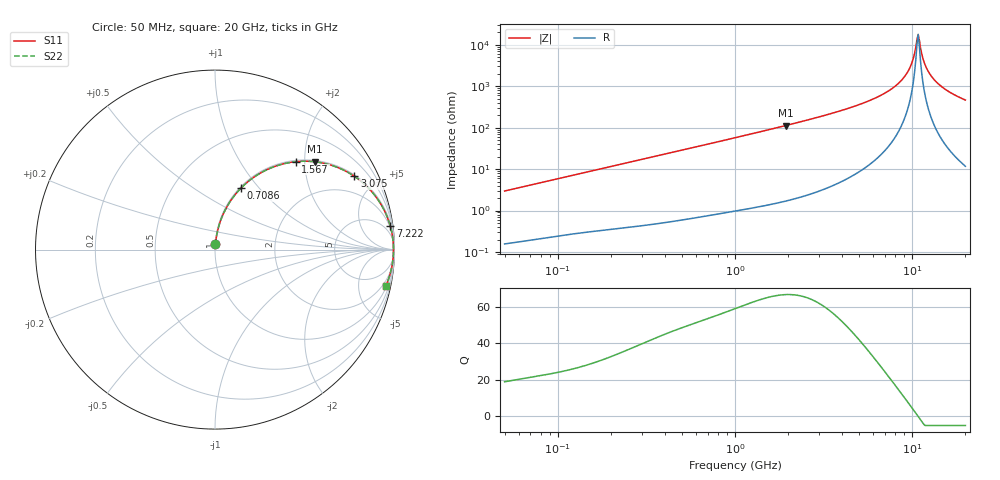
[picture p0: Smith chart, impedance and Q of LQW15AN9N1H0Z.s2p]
!Murata Part Number: LQW15AN9N1H0Z
!These Parameters are Measured in Series Mode Connection
!  o--[Z]--o
!Port1  Port2
!  o-------o
!Freq. Start=50[MHz] Stop=20[GHz], 401[Steps]
# Hz S RI R 50
!Freq.(Hz) S11(Real) S11(Imag) S21(Real) S21(Imag) S12(Real) S12(Imag) S22(Real) S22(Imag)
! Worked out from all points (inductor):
!   401 points, 50 MHz to 20 GHz, reference 50 ohm
!   read as one part in series: L = 9.38 nH near 51.52 MHz
!   highest Q = 66.6 at 1.933 GHz (marker M1), where L = 9.27 nH
!   self-resonance near 10.66 GHz
!   S11 on the Smith chart (normalised r, x): 50 MHz: 1.00, +0.06; 708.6 MHz: 1.02, +0.81; 1.567 GHz: 1.03, +1.81; 3.075 GHz: 1.06, +3.77; 7.222 GHz: 2, +15; 20 GHz: 1.23, -9.29
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5e7  0.00243 0.0295  0.9976 -0.0295  0.9976 -0.0295  0.00243 0.0295
1.364002e8  0.00906 0.0781  0.9909 -0.0781  0.9909 -0.0781  0.00906 0.0781
3.721004e8  0.0476 0.2017  0.9524 -0.2017  0.9524 -0.2017  0.0476 0.2017
7.08568e8  0.1449 0.3428  0.8551 -0.3428  0.8551 -0.3428  0.1449 0.3428
1e9  0.2495 0.4243  0.7505 -0.4243  0.7505 -0.4243  0.2495 0.4243
1.567309e9  0.4501 0.4899  0.5499 -0.4899  0.5499 -0.4899  0.4501 0.4899
1.932977e9  0.558 0.4892  0.442 -0.4892  0.442 -0.4892  0.558 0.4892
2.728004e9  0.7259 0.4383  0.2741 -0.4383  0.2741 -0.4383  0.7259 0.4383
3.075291e9  0.7763 0.4086  0.2237 -0.4086  0.2237 -0.4086  0.7763 0.4086
5.117541e9  0.927 0.2482  0.073 -0.2482  0.073 -0.2482  0.927 0.2482
7.222371e9  0.9761 0.1323  0.0239 -0.1323  0.0239 -0.1323  0.9761 0.1323
7.442007e9  0.9788 0.1224  0.0212 -0.1224  0.0212 -0.1224  0.9788 0.1224
8.516016e9  0.9881 0.0779  0.0119 -0.0779  0.0119 -0.0779  0.9881 0.0779
9.457416e9  0.9924 0.0436  0.0076 -0.0436  0.0076 -0.0436  0.9924 0.0436
9.892087e9  0.9935 0.029  0.0065 -0.029  0.0065 -0.029  0.9935 0.029
1.050288e10  0.9943 0.0095  0.00571 -0.0095  0.00571 -0.0095  0.9943 0.0095
1.082228e10  0.9944 -0.000239  0.0056 0.000239  0.0056 0.000239  0.9944 -0.000239
1.115139e10  0.9943 -0.00998  0.00568 0.00998  0.00568 0.00998  0.9943 -0.00998
1.183995e10  0.9936 -0.0295  0.00643 0.0295  0.00643 0.0295  0.9936 -0.0295
1.314879e10  0.9904 -0.0637  0.00961 0.0637  0.00961 0.0637  0.9904 -0.0637
1.573793e10  0.9791 -0.123  0.0209 0.123  0.0209 0.123  0.9791 -0.123
2e10  0.951 -0.2035  0.049 0.2035  0.049 0.2035  0.951 -0.2035
